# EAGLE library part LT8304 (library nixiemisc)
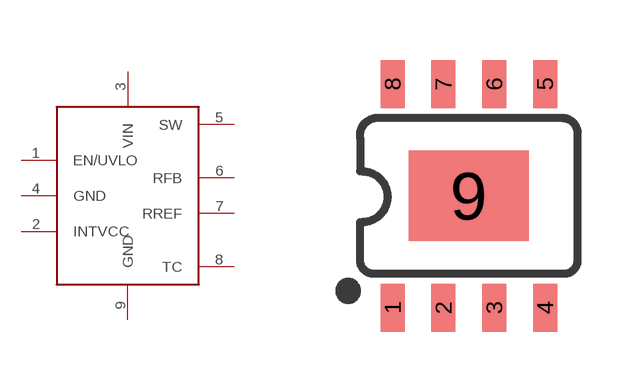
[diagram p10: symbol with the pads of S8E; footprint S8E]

Designator prefix U

## LT8304  [S8E]
1  EN/UVLO  pas
2  INTVCC  pas
3  VIN  pwr
4  GND  pwr
5  SW  pas
6  RFB  pas
7  RREF  pwr
8  TC  pas
9  GND  pwr

## Footprint S8E (pad centres in mm)
SOIC, 0.15 inch width
smd 0.6 x 1.2: 1 -1.905,-2.8; 2 -0.635,-2.8; 3 0.635,-2.8; 4 1.905,-2.8; 5 1.905,2.8; 6 0.635,2.8; 7 -0.635,2.8; 8 -1.905,2.8
smd 2.997 x 2.261: 9 0,0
